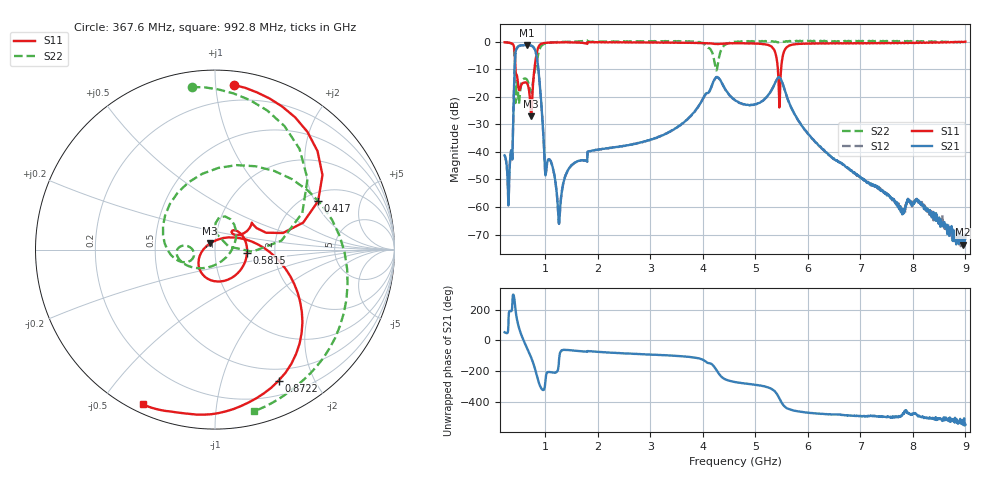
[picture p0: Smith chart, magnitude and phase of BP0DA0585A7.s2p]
!Agilent Technologies,E8358A,US41080443,A.07.50.56
!Agilent E8358A: A.07.50.56
!Date: Friday, November 10, 2017 15:00:12
!Correction: S11(Full 2 Port(1,2))
!S21(Full 2 Port(1,2))
!S12(Full 2 Port(1,2))
!S22(Full 2 Port(1,2))
!S2P File: Measurements: S11, S21, S12, S22:
# Hz S  dB  R 50
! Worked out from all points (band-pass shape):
!   1601 points, 225 MHz to 9 GHz, reference 50 ohm
!   highest |S21| = -1.25 dB at 652.8 MHz (marker M1); lowest = -73.7 dB at 8.956 GHz (marker M2)
!   |S21| within 3 dB of the highest: 432.1 MHz to 823.4 MHz (391.4 MHz wide, 62.3 % of centre)
!   lowest |S11| = -27.1 dB at 729.6 MHz (marker M3), VSWR 1.09, Z = 47.1 + j3.21 ohm
!   |S11| at or under -10 dB: 432.3 MHz to 791.8 MHz (359.5 MHz wide, 58.7 % of centre); 5.429 GHz to 5.49 GHz (61.23 MHz wide, 1.12 % of centre)
!   |S22| runs from -22.6 to 0.5 dB; largest |S21 - S12| = 0.0057
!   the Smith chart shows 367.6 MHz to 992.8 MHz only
!   S11 on the Smith chart (normalised r, x): 367.6 MHz: 0.09, +1.12; 417 MHz: 2.35, +2.12; 581.5 MHz: 1.43, -0.05; 872.2 MHz: 0.36, -1.54; 992.8 MHz: 0.04, -0.63
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2.25e8  -0.21 138.8  -41.27 53.1  -41.20 53.0  -0.17 149.4
3.675938e8  -0.69 83.5  -41.77 -149.6  -41.81 -149.5  -0.77 98.2
4.169531e8  -3.95 25.2  -9.14 -106.9  -9.19 -106.9  -5.55 22.8
4.992188e8  -17.47 39.7  -1.51 82.1  -1.55 82.0  -22.56 -59.7
5.814844e8  -14.93 -5.3  -1.28 4.1  -1.31 4.1  -13.58 -167.1
6.527812e8  -15.11 -92.1  -1.25 -50.0  -1.31 -50.1  -13.86 177.0
7.295625e8  -27.06 129.9  -1.39 -110.4  -1.44 -110.5  -18.48 -169.5
8.721562e8  -1.81 -64.1  -10.82 88.9  -10.85 89.0  -3.82 23.1
9.928125e8  -0.44 -115.1  -45.81 63.5  -45.77 63.4  -0.67 -76.5
1.261547e9  -0.27 -156.2  -66.13 -126.2  -66.05 -130.2  -0.11 -119.8
1.689328e9  -0.36 165.0  -43.02 -71.1  -43.10 -71.3  0.18 -126.5
3.153656e9  -0.28 144.7  -34.52 -94.9  -34.59 -95.1  0.21 -150.4
3.987281e9  -0.48 121.9  -21.16 -123.4  -21.23 -123.6  -0.40 -168.5
4.212141e9  -0.75 115.3  -14.06 -170.3  -14.12 -170.0  -6.41 123.5
4.310859e9  -0.80 114.5  -13.39 140.4  -13.44 139.7  -5.46 -41.1
4.6125e9  -0.58 105.4  -21.23 88.3  -21.20 88.5  -0.05 -114.5
5.22675e9  -1.10 74.1  -19.82 55.5  -19.90 54.9  0.09 -131.0
5.457094e9  -23.87 -66.2  -12.90 -18.5  -12.90 -18.6  -0.15 -133.4
6.076828e9  -0.66 82.0  -35.10 -113.8  -35.11 -114.1  0.17 -141.5
7.541156e9  -0.43 42.0  -55.94 -139.7  -56.16 -141.9  0.16 -155.1
8.956125e9  -0.12 33.1  -73.72 -174.6  -73.98 177.4  -0.17 -175.4
9e9  0.01 33.3  -69.85 170.2  -70.40 -178.8  -0.25 -176.5
